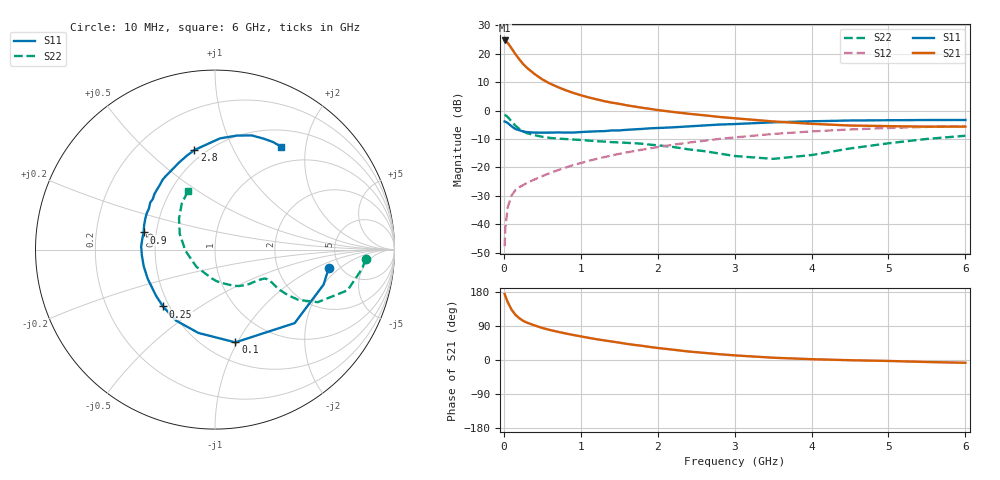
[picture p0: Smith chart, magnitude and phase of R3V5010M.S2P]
! SIEMENS Small Signal Semiconductors
! BFR181
! Si NPN RF Bipolar Junction Transistor in SOT23
! VCE = 0.5 V  IC = 10 mA
! Common Emitter S-Parameters:  May  1996
# GHz  S  MA  R  50
!  f  S11  S21  S12  S22
! GHz  MAG  ANG  MAG  ANG  MAG  ANG  MAG  ANG
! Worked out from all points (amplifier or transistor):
!   36 points, 10 MHz to 6 GHz, reference 50 ohm
!   highest |S21| = 24.7 dB at 10 MHz (marker M1)
!   |S21| within 3 dB of that: start of sweep to 106.1 MHz
!   unconditionally stable (mu >= 1): start of sweep to 13.23 MHz; 232.8 MHz to end of sweep
!   at 250 MHz: K = 1.06, MAG = 19.9 dB, |S12| = -26.2 dB
!   at 1.4 GHz: K = 1.64, MAG = 4.6 dB, |S12| = -15.8 dB
!   at 6 GHz: K = 1.22, MAG = -2.9 dB, |S12| = -5.5 dB
!   S11 on the Smith chart (normalised r, x): 10 MHz: 4.04, -1.44; 100 MHz: 0.68, -0.98; 250 MHz: 0.46, -0.36; 900 MHz: 0.42, +0.10; 2.8 GHz: 0.44, +0.72; 6 GHz: 0.74, +1.58
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0.01  0.6418 -9.4  17.12 174.3  0.0041 83.1  0.8412 -3.7
0.02  0.6357 -17.9  16.85 168.4  0.0086 76.0  0.8263 -7.4
0.05  0.6039 -42.7  15.56 152.9  0.0197 69.4  0.7726 -17.1
0.1  0.5291 -77.6  12.47 132.9  0.0319 58.6  0.6429 -27.1
0.15  0.4736 -101.2  9.841 119.4  0.0398 52.9  0.5428 -31.1
0.2  0.4511 -118.6  7.997 110.4  0.0447 51.2  0.4762 -32.0
0.25  0.4294 -132.5  6.611 103.5  0.0487 50.8  0.4297 -31.9
0.3  0.4169 -142.1  5.659 98.6  0.0532 52.0  0.4002 -31.3
0.4  0.4087 -156.4  4.385 91.2  0.0613 54.4  0.3678 -30.1
0.5  0.4079 -166.9  3.53 84.5  0.07 56.2  0.3453 -29.6
0.6  0.4087 -175.6  2.981 79.2  0.0795 58.0  0.3299 -29.7
0.7  0.4117 177.7  2.597 74.5  0.0889 59.4  0.3206 -30.2
0.9  0.4092 166.5  2.049 66.1  0.1092 60.5  0.3098 -32.1
1.1  0.4247 156.3  1.708 58.6  0.13 61.1  0.2961 -35.3
1.3  0.4336 148.1  1.468 51.9  0.1509 60.6  0.2846 -38.9
1.6  0.4582 137.4  1.234 42.5  0.1838 59.1  0.2698 -45.3
2.2  0.5061 118.0  0.944 27.2  0.2499 53.8  0.2285 -62.2
2.8  0.5663 101.7  0.772 15.3  0.3165 46.7  0.1752 -87.7
3.5  0.6204 87.4  0.643 6.0  0.387 37.2  0.141 -137.5
4.5  0.6681 72.2  0.545 -0.6  0.4642 22.8  0.2151 156.0
5.5  0.681 61.7  0.52 -5.3  0.5155 9.8  0.3165 125.8
6  0.6816 57.2  0.521 -7.3  0.533 3.4  0.3597 114.6
